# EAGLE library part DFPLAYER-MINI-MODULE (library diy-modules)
DFPlayer Mini - MP3 player module based on YX5200 chip More details available here: https://www.dfrobot.com/wiki/index.php/DFPlayer_Mini_SKU:DFR0299 Click here to find device on ebay.com
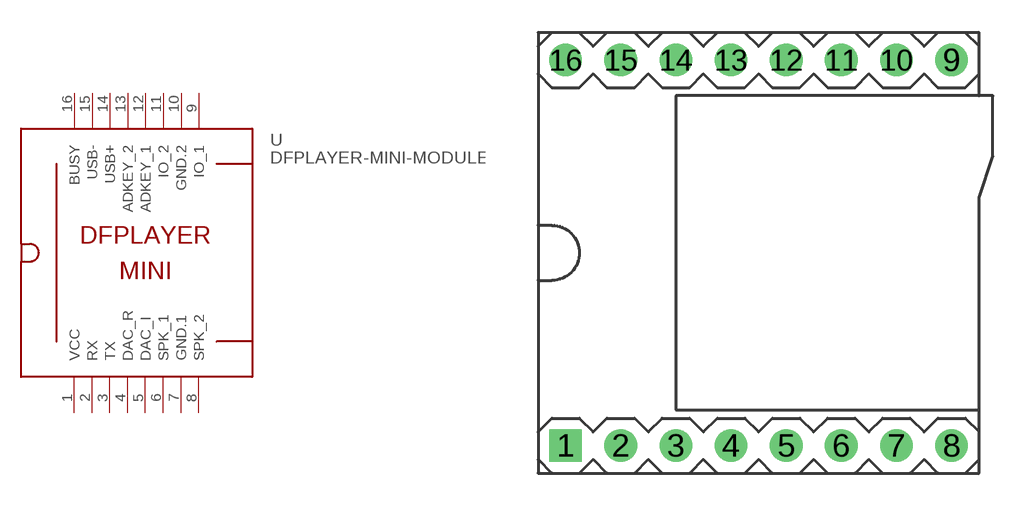
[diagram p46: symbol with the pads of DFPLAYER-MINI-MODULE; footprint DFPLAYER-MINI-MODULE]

Designator prefix -

## DFPLAYER-MINI-MODULE  [DFPLAYER-MINI-MODULE]
1  VCC  pwr
2  RX
3  TX
4  DAC_R
5  DAC_I
6  SPK_1
7  GND.1  pwr
8  SPK_2
9  IO_1
10  GND.2  pwr
11  IO_2
12  ADKEY_1
13  ADKEY_2
14  USB+
15  USB-
16  BUSY

## Footprint DFPLAYER-MINI-MODULE (pad centres in mm)
DFPlayer Mini - MP3 player module based on YX5200 chip
drill 1 square: 1 -8.89,-8.89
drill 1: 2 -6.35,-8.89; 3 -3.81,-8.89; 4 -1.27,-8.89; 5 1.27,-8.89; 6 3.81,-8.89; 7 6.35,-8.89; 8 8.89,-8.89; 9 8.89,8.89; 10 6.35,8.89; 11 3.81,8.89; 12 1.27,8.89; 13 -1.27,8.89; 14 -3.81,8.89; 15 -6.35,8.89; 16 -8.89,8.89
